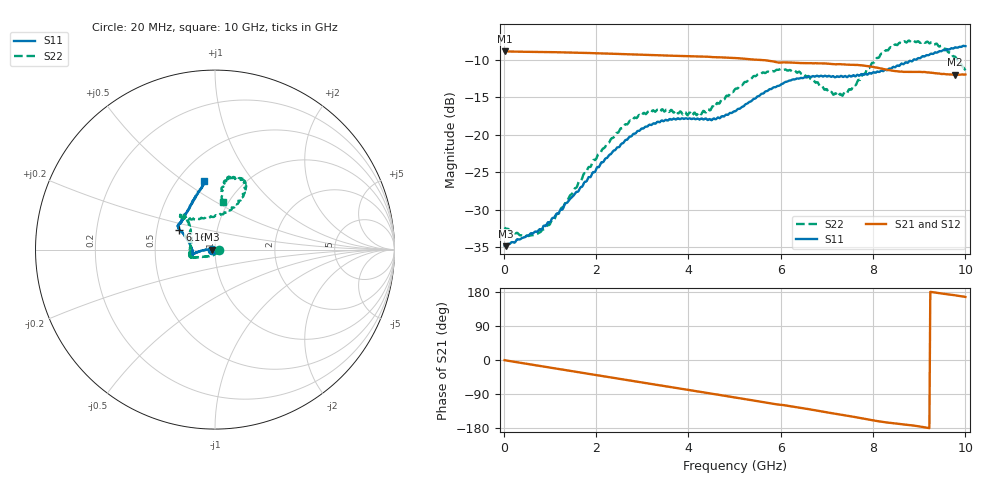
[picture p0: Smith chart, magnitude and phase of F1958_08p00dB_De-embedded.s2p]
! Integrated Device Technology
! Corporate Headquarters
! 6024 Silver Creek Valley Road
! San Jose, CA 95138  USA
! Phone:  1-408-284-8200
! Toll Free:  1-800-223-1366
! Webpage:  http://www.idt.com/
! Timing and RF Division
! 515 Groton Road, Suite 102
! Westford, MA 01886-6024
! Device:  F1958
! Description: 7-bit 0.25 dB Digital Step Attenuator
! Frequency:  0.001 -  6.000 GHz
! Package:  4x4 mm Thin QFN Plastic Package: 24 pin
! Ports:  2 RF, 12 DC
!  Pin  1  = D0
!  Pin  2  = VDD
!  Pin  3  = VMODE
!  Pin  4  = GND
!  Pin  5  = RF1  =  Port 1
!  Pin  6  = GND
!  Pin  7  = GND
!  Pin  8  = GND
!  Pin  9  = GND
!  Pin 10  = GND
!  Pin 11  = GND
!  Pin 12  = GND
!  Pin 13  = GND
!  Pin 14  = RF2  =  Port 2
!  Pin 15  = GND
!  Pin 16  = LE
!  Pin 17  = CLK
!  Pin 18  = DATA
!  Pin 19  = D6
!  Pin 20  = D5
!  Pin 21  = D4
!  Pin 22  = D3
!  Pin 23  = D2
!  Pin 24  = D1
! State:  32
! Atten State:  8.00 dB
! Voltage:  +3.30 Volts
! Current:  0.258 mA
! Data:  The device was measured on a F1958 evaluation board which has
!  individual transmission lines to the RF pins.  Data was collected
!  using a calibrated network analyzer.  The evaluation board was
!  de-embedded using Automatic Fixture Removal (AFR).
!  The reference plane is the edge of the package pin.
! Misc:
!  Action Tracker AT0419
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# GHz S dB R 50
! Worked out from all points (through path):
!   500 points, 20 MHz to 10 GHz, reference 50 ohm
!   highest |S21| = -8.90 dB at 20 MHz (marker M1); lowest = -12.0 dB at 9.78 GHz (marker M2)
!   group delay of S21, straight-line fit = 54.3 ps
!   lowest |S11| = -34.8 dB at 40 MHz (marker M3), VSWR 1.04, Z = 48.2 - j0.0842 ohm
!   |S11| at or under -10 dB: start of sweep to 8.879 GHz; 8.917771 GHz to 8.92744 GHz (9.67 MHz wide, 0.108 % of centre)
!   |S22| runs from -33.6 to -7.5 dB; largest |S21 - S12| = 0.001
!   S11 on the Smith chart (normalised r, x): 20 MHz: 0.96, -0.00; 6.16 GHz: 0.65, +0.15; 10 GHz: 0.67, +0.60
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0.02  -34.77 -177.6  -8.90 -0.5  -8.90 -0.5  -32.32 -5.4
0.04  -34.83 -177.2  -8.91 -0.9  -8.90 -0.9  -32.49 -8.3
0.44  -33.66 174.8  -8.96 -8.9  -8.96 -8.9  -33.60 -34.3
0.76  -32.67 175.4  -8.98 -15.2  -8.98 -15.2  -33.06 -62.1
1.1  -30.98 178.2  -9.01 -22.0  -9.01 -22.0  -31.26 -94.9
1.7  -26.91 -178.2  -9.10 -33.8  -9.10 -33.7  -25.79 -135.3
2.6  -21.03 -172.9  -9.28 -51.5  -9.26 -51.5  -18.94 -158.2
2.94  -19.47 -170.6  -9.35 -58.2  -9.33 -58.3  -17.35 -160.5
3.36  -18.32 -168.4  -9.44 -66.4  -9.44 -66.5  -16.83 -164.5
4.24  -17.99 -172.5  -9.59 -83.6  -9.60 -83.7  -17.03 166.6
5.02  -16.86 167.7  -9.79 -99.1  -9.81 -99.2  -13.87 136.0
5.54  -14.81 156.2  -10.04 -109.5  -10.05 -109.5  -11.92 132.8
6.16  -12.87 150.6  -10.37 -121.1  -10.39 -121.0  -11.47 135.6
6.68  -12.23 147.4  -10.49 -131.2  -10.50 -131.1  -12.60 131.6
7.1  -12.30 143.4  -10.59 -140.2  -10.59 -140.1  -14.30 113.0
7.34  -12.29 142.0  -10.63 -145.1  -10.64 -144.9  -14.80 92.5
7.9  -11.88 130.7  -10.87 -157.1  -10.87 -157.1  -11.12 65.9
8.34  -11.22 121.1  -11.40 -165.5  -11.40 -165.6  -8.64 62.7
8.76  -10.39 112.1  -11.65 -171.3  -11.66 -171.3  -7.51 67.7
9.24  -9.25 103.8  -11.75 179.8  -11.75 179.8  -7.81 77.8
9.78  -8.38 99.2  -12.02 170.6  -12.04 170.6  -9.62 83.0
10  -8.21 98.8  -11.98 166.3  -12.00 166.5  -11.43 80.6
